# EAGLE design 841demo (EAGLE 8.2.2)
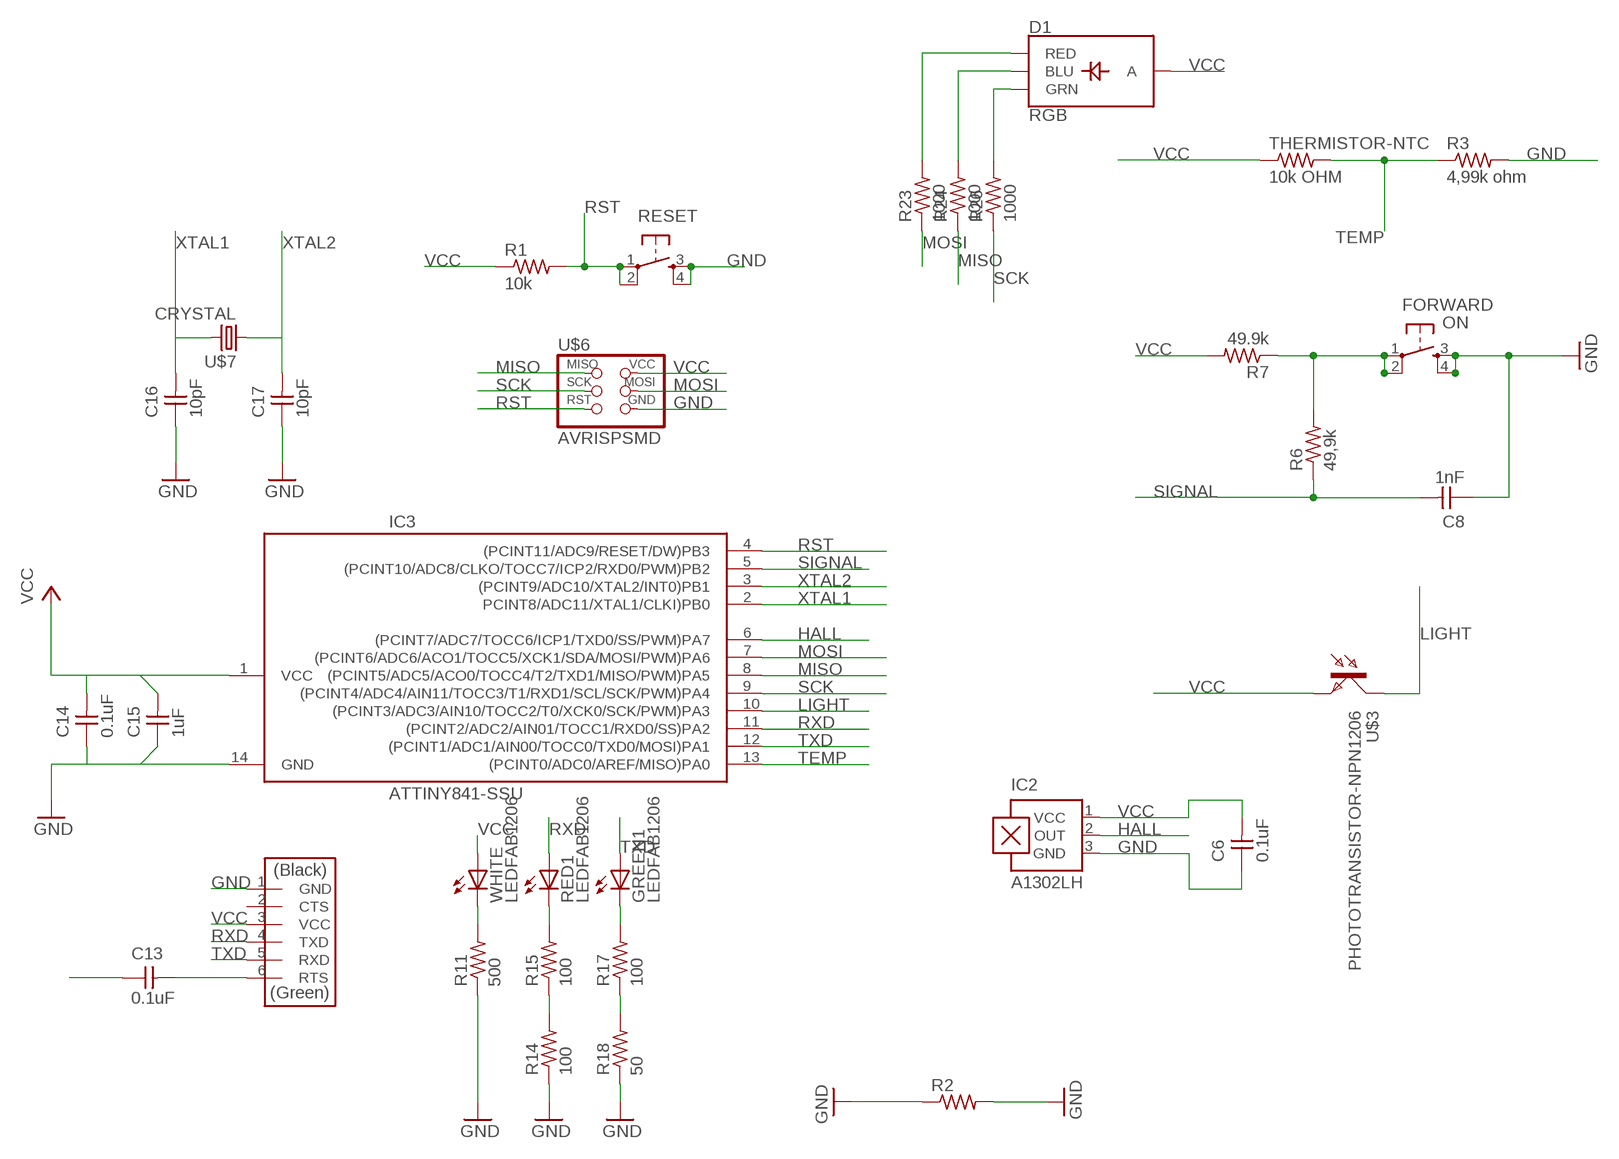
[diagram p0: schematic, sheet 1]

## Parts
C6  0.1uF  CAP-UNPOLARIZEDFAB  [C1206FAB]
C8  1nF  CAP-UNPOLARIZEDFAB  [C1206FAB]
C13  0.1uF  CAP-UNPOLARIZEDFAB  [C1206FAB]
C14  0.1uF  CAP-UNPOLARIZEDFAB  [C1206FAB]
C15  1uF  CAP-UNPOLARIZEDFAB  [C1206FAB]
C16  10pF  CAP-UNPOLARIZEDFAB  [C1206FAB]
C17  10pF  CAP-UNPOLARIZEDFAB  [C1206FAB]
D1  RGB  LED-RGB-CAPLCC  [P-LCC-4-3]
FORWARD  ON  6MM_SWITCH6MM_SWITCH  [6MM_SWITCH]
GREEN1  LEDFAB1206  [LED1206FAB]
IC2  A1302LH  [SOT23-W]
IC3  ATTINY841-SSU  [SOIC14]
R1  10k  RES-US1206FAB  [R1206FAB]
R2  RES-US1206FAB  [R1206FAB]
R3  4,99k ohm  RES-US1206FAB  [R1206FAB]
R6  49,9k  RES-US1206FAB  [R1206FAB]
R7  49.9k  RES-US1206FAB  [R1206FAB]
R11  500  RES-US1206FAB  [R1206FAB]
R14  100  RES-US1206FAB  [R1206FAB]
R15  100  RES-US1206FAB  [R1206FAB]
R17  100  RES-US1206FAB  [R1206FAB]
R18  50  RES-US1206FAB  [R1206FAB]
R23  1000  RES-US1206FAB  [R1206FAB]
R24  1000  RES-US1206FAB  [R1206FAB]
R26  1000  RES-US1206FAB  [R1206FAB]
RED1  LEDFAB1206  [LED1206FAB]
RESET  6MM_SWITCH6MM_SWITCH  [6MM_SWITCH]
SERIAL1  FTDI-SMD-HEADER  [1X06SMD]
THERMISTOR-NTC  10k OHM  RES-US1206FAB  [R1206FAB]
U$3  PHOTOTRANSISTOR-NPN1206  [OP1206]
U$6  AVRISPSMD  [2X03SMD]
U$7  CRYSTAL  [2-SMD-5X3MM]
WHITE  LEDFAB1206  [LED1206FAB]

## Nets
GND: C6.1 C8.1 C14.1 C15.1 C16.1 C17.1 FORWARD.3(S) FORWARD.4(S1) IC2.3(GND) IC3.14(GND) R2.1 R2.2 R3.2 R11.1 R14.1 R18.1 RESET.3(S) RESET.4(S1) SERIAL1.1(GND) U$6.6(GND)
HALL: IC2.2(OUT) IC3.6((PCINT7/ADC7/TOCC6/ICP1/TXD0/SS/PWM)PA7)
LIGHT: IC3.10((PCINT3/ADC3/AIN10/TOCC2/T0/XCK0/SCK/PWM)PA3) U$3.COLLECTOR(C)
MISO: IC3.8((PCINT5/ADC5/ACO0/TOCC4/T2/TXD1/MISO/PWM)PA5) R24.1 U$6.1(MISO)
MOSI: IC3.7((PCINT6/ADC6/ACO1/TOCC5/XCK1/SDA/MOSI/PWM)PA6) R23.1 U$6.4(MOSI)
N$1: FORWARD.1(P) FORWARD.2(P1) R6.2 R7.1
N$2: R15.2 RED1.2(C)
N$3: R17.1 R18.2
N$4: R14.2 R15.1
N$5: GREEN1.2(C) R17.2
N$6: D1.3(BLU) D1.L3(BLU) R24.2
N$7: D1.2(GRN) D1.L2(GRN) R26.2
N$8: R11.2 WHITE.2(C)
N$9: D1.1(RED) D1.L1(RED) R23.2
N$11: C13.2 SERIAL1.6(RTS)
RST: C13.1 IC3.4((PCINT11/ADC9/RESET/DW)PB3) R1.2 RESET.1(P) RESET.2(P1) U$6.5(RST)
RXD: IC3.11((PCINT2/ADC2/AIN01/TOCC1/RXD0/SS)PA2) RED1.1(A) SERIAL1.4(TXD)
SCK: IC3.9((PCINT4/ADC4/AIN11/TOCC3/T1/RXD1/SCL/SCK/PWM)PA4) R26.1 U$6.3(SCK)
SIGNAL: C8.2 IC3.5((PCINT10/ADC8/CLKO/TOCC7/ICP2/RXD0/PWM)PB2) R6.1
TEMP: IC3.13((PCINT0/ADC0/AREF/MISO)PA0) R3.1 THERMISTOR-NTC.2
TXD: GREEN1.1(A) IC3.12((PCINT1/ADC1/AIN00/TOCC0/TXD0/MOSI)PA1) SERIAL1.5(RXD)
VCC: C6.2 C14.2 C15.2 D1.4(A) D1.L4(A) IC2.1(VCC) IC3.1(VCC) R1.1 R7.2 SERIAL1.3(VCC) THERMISTOR-NTC.1 U$3.EMITTER(E) U$6.2(VCC) WHITE.1(A)
XTAL1: C16.2 IC3.2(PCINT8/ADC11/XTAL1/CLKI)PB0) U$7.P$2
XTAL2: C17.2 IC3.3((PCINT9/ADC10/XTAL2/INT0)PB1) U$7.P$1
Unconnected: SERIAL1.2(CTS)

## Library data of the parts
C6 C8 C13-C17 = fab:CAP-UNPOLARIZED
D1 = chrysi:LED-RGB-CA: LED-RGB Diffused Common Anode Packages: LED RGB-THRU P-LCC-4-3 LED-TRICOLOR-SMD SparkFun Products: RGB Diffused Common Anode- Diffuse RGB Diffused Common Anode - Clear Qduino Mini Triple Output LED RGB - SMD; PROD_ID: DIO-12986
FORWARD RESET = fab:6MM_SWITCH: OMRON SWITCH
GREEN1 RED1 WHITE = fab:LED: LED
IC2 = allegro:A13*?: Linear Hall Effect Sensor ICs Continuous-Time Ratiometric High-Temperature Operation Programmable Linear with Analog Output A1302 -Replacement- UGN3503 Source: http://www.allegromicro.com/en/Products/Part_Numbers/1301/1301.pdf http://www.allegromicro.com/en/Products/Part_Numbers/1321/1321.pdf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; MF: ALLEGRO MICROSYSTEMS, INC.; MPN: A1302ELHLT-T; OC_FARNELL: 1457209; OC_NEWARK: 31K6638
IC3 = chrysi:ATTINY841: For Arduino usage https://github.com/SpenceKonde/ATTinyCore Datasheet http://www.atmel.com/Images/Atmel-8495-8-bit-AVR-Microcontrollers-ATtiny441-ATtiny841_Datasheet.pdf
R1-R3 R6 R7 R11 R14 R15 R17 R18 R23 R24 R26 THERMISTOR-NTC = fab:RES-US: Resistor (US Symbol)
SERIAL1 = fab:FTDI-SMD-HEADER
U$3 = fab:PHOTOTRANSISTOR-NPN
U$6 = fab:AVRISP
U$7 = fab:CRYSTAL

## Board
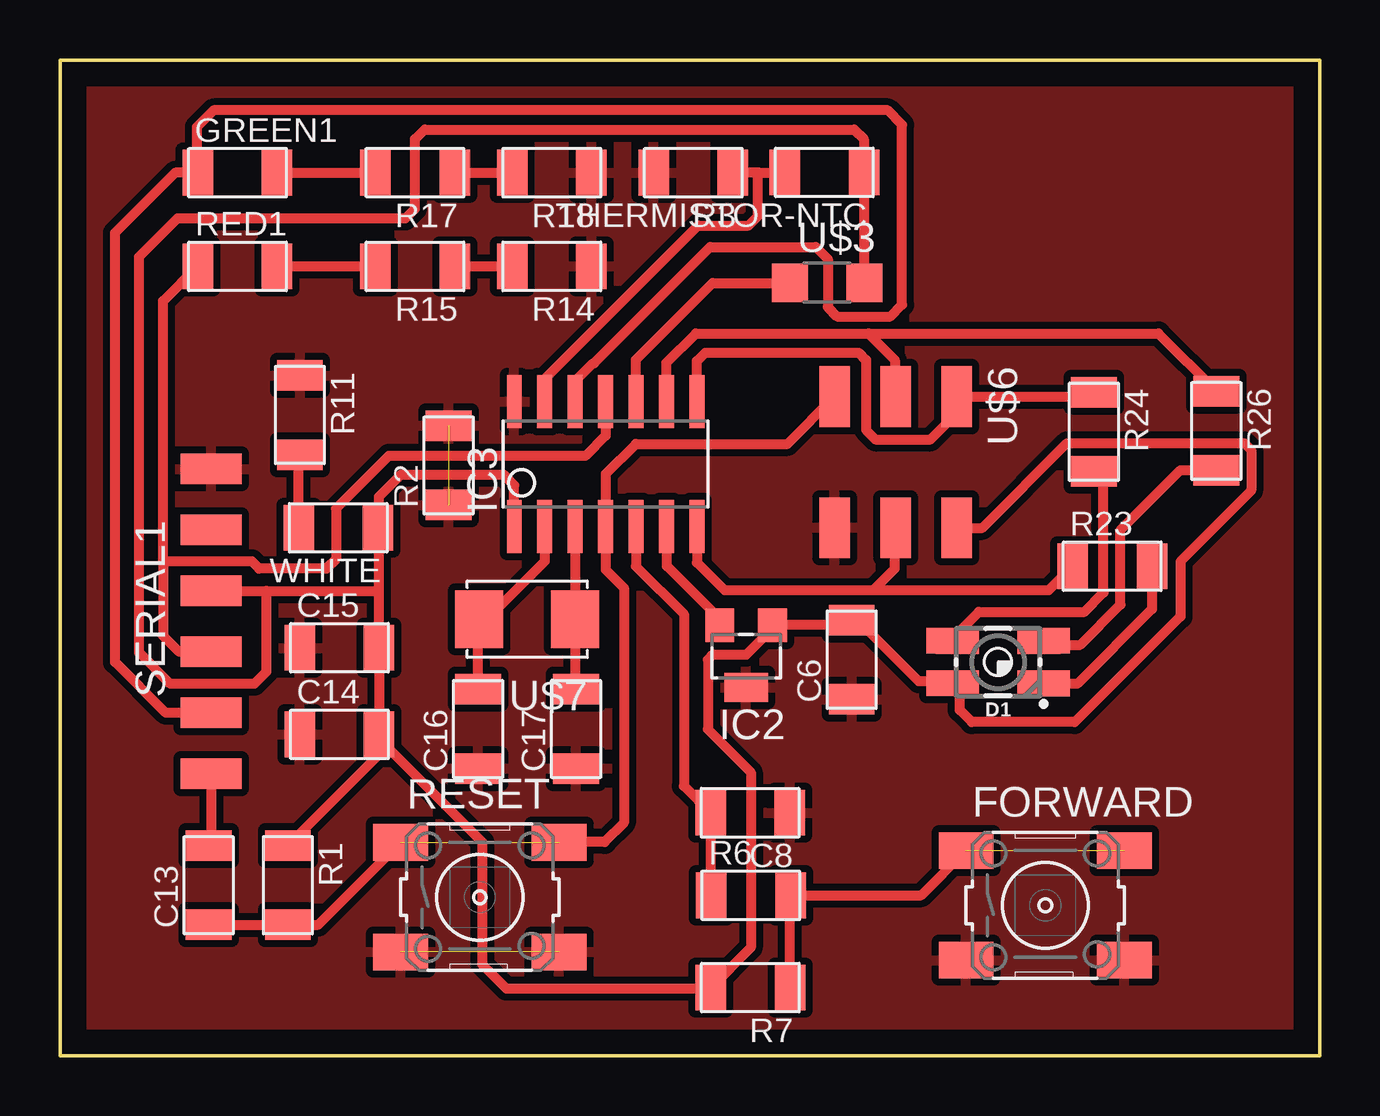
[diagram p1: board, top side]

Size 52.5 x 41.5 mm. Coordinates in mm from the lower left corner, seen from the top.
Outline: 0,0 52.5,0 52.5,41.5 0,41.5 0,0
Copper layers (1*16): Top 0.035mm / dielectric 1.5mm / Bottom 0.035mm
Design rules "Chrysi": minimum track width 0.3mm, minimum drill 0.6mm, track to track 0.3mm, track to pad 0.3mm, pad to pad 0.3mm, via to via 0.3mm, smd to smd 0.3mm, copper to edge 40mil, drill to drill 8mil, minimum pad ring 10mil, minimum via ring 8mil, stop-mask expansion 4mil, vias tented up to drill 0mil, thermal gap 0.3mm

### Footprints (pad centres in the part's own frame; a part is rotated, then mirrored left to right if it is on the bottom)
C1206FAB = smd 1.27 x 1.905: 1 -1.651,0; 2 1.651,0
P-LCC-4-3 = smd 1.8 x 0.75: 1 -1.7,0.725; 2 -1.7,-0.725; 3 1.7,-0.725; 4 1.7,0.725 | smd 2.184 x 1.067: L1 -1.893,0.89; L2 -1.893,-0.884; L3 1.892,-0.884; L4 1.892,0.884
6MM_SWITCH = smd 2.286 x 1.524: 1 -3.302,2.286; 2 3.302,2.286; 3 -3.302,-2.286; 4 3.302,-2.286
LED1206FAB = smd 1.27 x 1.905: 1 -1.651,0; 2 1.651,0
SOT23-W = smd 1.2 x 1.4: 1 -1.1,-1.3; 2 1.1,-1.3 | smd 1.8 x 1.2: 3 0,1.3
SOIC14 = smd 0.61 x 2.21: 1 -3.81,-2.603; 2 -2.54,-2.603; 3 -1.27,-2.603; 4 0,-2.603; 5 1.27,-2.603; 6 2.54,-2.603; 7 3.81,-2.603; 8 3.81,2.603; 9 2.54,2.603; 10 1.27,2.603; 11 0,2.603; 12 -1.27,2.603; 13 -2.54,2.603; 14 -3.81,2.603
R1206FAB = smd 1.27 x 1.905: 1 -1.651,0; 2 1.651,0
1X06SMD = smd 2.54 x 1.27: 1 0,6.35; 2 0,3.81; 3 0,1.27; 4 0,-1.27; 5 0,-3.81; 6 0,-6.35
OP1206 = smd 1.5 x 1.6: COLLECTOR -1.55,0; EMITTER 1.55,0
2X03SMD = smd 2.54 x 1.27: 1 -2.54,2.54; 2 2.92,2.54; 3 -2.54,0; 4 2.92,0; 5 -2.54,-2.54; 6 2.92,-2.54
2-SMD-5X3MM = smd 2 x 2.4: P$1 -2,0; P$2 2,0

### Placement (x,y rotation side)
C6  33,16.5 90 top
C8  28.77,10.12 180 top
C13  6.2,7.1 90 top
C14  11.65,13.39 0 top
C15  11.65,17 0 top
C16  17.43,13.61 90 top
C17  21.51,13.61 90 top
D1  39.1,16.4 180 top
FORWARD  41.07,6.26 0 top
GREEN1  7.4,36.8 0 top
IC2  28.6,16.64 180 top
IC3  22.74,24.65 0 top
R1  9.5,7.1 270 top
R2  16.2,24.6 90 top
R3  26.4,36.8 180 top
R6  28.8,6.68 0 top
R7  28.78,2.83 180 top
R11  10,26.7 270 top
R14  20.5,32.9 180 top
R15  14.8,32.9 180 top
R17  14.8,36.8 180 top
R18  20.5,36.8 180 top
R23  43.86,20.4 0 top
R24  43.09,26 270 top
R26  48.2,26.04 270 top
RED1  7.4,32.9 0 top
RESET  17.5,6.6 0 top
SERIAL1  6.3,18.1 0 top
THERMISTOR-NTC  31.86,36.81 180 top
U$3  31.98,32.21 0 top
U$6  34.83,24.92 270 top
U$7  19.47,18.19 180 top
WHITE  11.6,22 180 top

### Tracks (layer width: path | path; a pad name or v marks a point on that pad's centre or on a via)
GND  (2 unrouted)
  pour Top: 0,0 52.5,0 52.5,41.5 0,41.5
HALL
  Top 0.406: IC2.2 27.5,18.2 25.3,20.4 25.3,22.03 IC3.6
LIGHT
  Top 0.406: IC3.10 24.01,29.01 27.2,32.2 U$3.COLLECTOR
MISO
  Top 0.406: R24.1 42.9,27.46 U$6.1 37.1,27.19 37.1,26.5 36.29,25.69 33.99,25.69 33.6,26.07 33.6,29 33.3,29.3 26.9,29.3 26.55,28.95 IC3.8
MOSI
  Top 0.406: IC3.7 26.55,20.55 27.7,19.4 33.9,19.4 | 33.9,19.4 34.8,20.3 34.8,21.97 U$6.4 | 33.9,19.4 41.21,19.4 R23.1
N$1  (1 unrouted)
  Top 0.406: R7.1 30.43,6.66 R6.2 35.9,6.68 FORWARD.1
N$2
  Top 0.406: RED1.2 R15.2
N$3
  Top 0.406: R17.1 R18.2
N$4
  Top 0.406: R15.1 R14.2
N$5
  Top 0.406: GREEN1.2 R17.2
N$6
  Top 0.406: D1.L3 37.37,17.12 D1.3 37.4,17.6 38.3,18.5 42.7,18.5 43.49,19.29 43.49,23.95 R24.2
N$7
  Top 0.406: D1.L2 40.84,17.12 D1.2 42.52,17.12 44.2,18.8 44.2,21.9 46.7,24.4 R26.2
N$8
  Top 0.406: WHITE.2 9.95,25 R11.2
N$9
  Top 0.406: 40.97,15.51 D1.L1 | 40.97,15.51 D1.1 | R23.2 45.51,18.61 42.4,15.5 40.98,15.5 40.97,15.51
N$11
  Top 0.406: SERIAL1.6 6.3,8.85 C13.2
RST  (1 unrouted)
  Top 0.406: C13.1 R1.2 10.76,5.45 RESET.1 | U$6.5 30.33,25.5 24,25.5 22.74,24.24 IC3.4 22.74,20.26 23.5,19.5 23.5,9.7 22.7,8.9 20.82,8.9 RESET.2
RXD
  Top 0.406: SERIAL1.4 4.97,16.83 4.3,17.5 4.3,20.55 | 4.3,20.55 4.3,31.45 RED1.1 | IC3.11 22.74,25.84 21.9,25 13.7,25 11.5,22.8 11.5,20.7 11.1,20.3 8.3,20.3 8,20.6 4.35,20.6 4.3,20.55
SCK
  Top 0.406: IC3.9 25.28,28.88 26.5,30.1 33.7,30.1 | 33.7,30.1 34.8,29 34.8,27.49 U$6.3 | 33.7,30.1 45.79,30.1 R26.1
SIGNAL
  Top 0.406: 27.02,6.55 R6.1 27.12,6.71 C8.2 26,11.24 26,18.4 24.01,20.39 IC3.5
TEMP
  Top 0.406: 29.18,36.8 R3.1 | 29.18,36.8 THERMISTOR-NTC.2 | IC3.13 20.2,28.2 26.6,34.6 28.7,34.6 29.1,35 29.1,36.72 29.18,36.8
TXD
  Top 0.406: SERIAL1.5 4.41,14.29 2.3,16.4 2.3,34.3 4.8,36.8 GREEN1.1 5.7,36.85 5.7,38.7 6.4,39.4 34.5,39.4 35.1,38.8 35.1,31.3 34.61,30.81 32.39,30.81 32,31.2 32,33.2 31.5,33.7 27.1,33.7 22.26,28.86 22.23,28.86 21.47,28.11 IC3.12
VCC
  Top 0.406: 37.18,15.6 35.8,15.6 33.25,18.15 C6.2 32.79,17.94 IC2.1 29.7,17.8 28.6,16.7 27.2,16.7 27,16.5 27,13.6 28.8,11.8 28.8,4.5 R7.2 27.1,2.8 18.6,2.8 17.6,3.8 17.6,8.9 13.3,13.2 C14.2 | 37.4,15.6 37.61,15.6 | 37.4,15.6 37.18,15.6 | 37.61,15.6 37.85,15.6 | IC3.1 18.93,23.77 18.5,24.2 14.2,24.2 13.3,23.3 13.3,22.05 | 13.3,22.05 WHITE.1 | 13.3,19.47 C15.2 C14.2 | 13.3,19.47 13.3,22.05 | SERIAL1.3 8.6,19.37 | 8.6,19.37 13.2,19.37 13.3,19.47 | U$3.EMITTER 33.53,36.79 THERMISTOR-NTC.1 33.5,38.2 33.1,38.6 15.2,38.6 14.8,38.2 14.8,35.3 14.4,34.9 4.9,34.9 3.3,33.3 3.3,16.8 4.6,15.5 8.1,15.5 8.6,16 8.6,19.37 | C14.2 13.3,12.55 R1.1 | D1.L4 37.21,15.57 37.18,15.6 | 37.41,15.52 D1.L4 | 37.41,15.52 37.53,15.52 37.61,15.6 | D1.L4 37.31,15.52 37.4,15.6 | D1.L4 37.24,15.52 D1.4 | U$6.2 38.44,22 41.97,25.53 49.36,25.53 49.66,25.23 49.66,23.55 46.7,20.59 46.7,18.3 42.3,13.9 38,13.9 37.5,14.4 37.5,15.43 37.41,15.52
XTAL1
  Top 0.406: IC3.2 20.2,20.6 18.1,18.5 17.78,18.5 U$7.P$2 17.43,18.15 C16.2
XTAL2
  Top 0.406: IC3.3 U$7.P$1 21.47,15.3 C17.2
